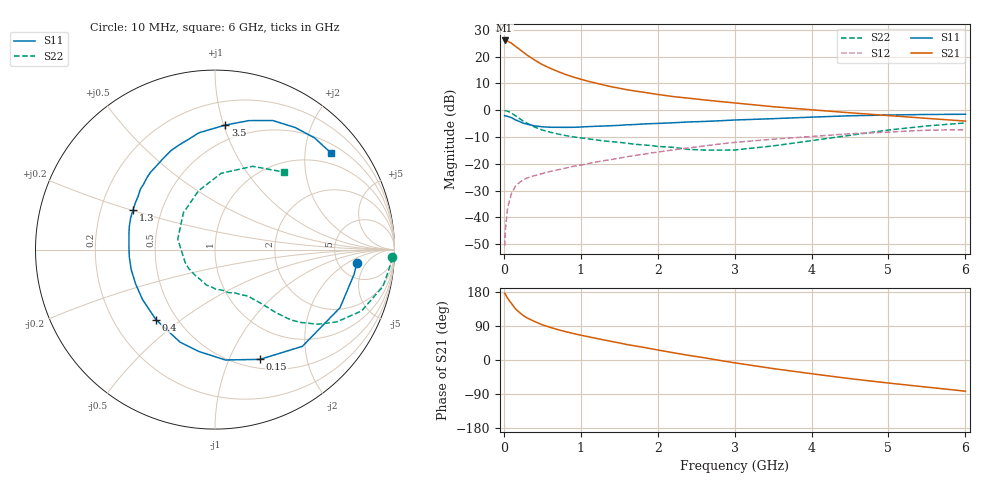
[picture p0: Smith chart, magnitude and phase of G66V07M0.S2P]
! SIEMENS Small Signal Semiconductors
! BFG193
! Si NPN RF Bipolar Junction Transistor in SOT223
! VCE = 6 V  IC = 7 mA
! Common Emitter S-Parameters:  August  1996
# GHz  S  MA  R  50
!  f  S11  S21  S12  S22
! GHz  MAG  ANG  MAG  ANG  MAG  ANG  MAG  ANG
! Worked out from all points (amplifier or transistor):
!   36 points, 10 MHz to 6 GHz, reference 50 ohm
!   highest |S21| = 26.0 dB at 10 MHz (marker M1)
!   |S21| within 3 dB of that: start of sweep to 189.6 MHz
!   unconditionally stable (mu >= 1): 1.019 GHz to 2.538 GHz
!   at 250 MHz: K = 0.42, MSG = 23.9 dB, |S12| = -26.0 dB
!   at 1.4 GHz: K = 1.08, MAG = 11.9 dB, |S12| = -18.4 dB
!   at 6 GHz: K = 0.86, MSG = 1.6 dB, |S12| = -7.3 dB
!   S11 on the Smith chart (normalised r, x): 10 MHz: 7.51, -2.98; 150 MHz: 0.60, -1.31; 400 MHz: 0.39, -0.41; 1.3 GHz: 0.34, +0.20; 3.5 GHz: 0.38, +1.01; 6 GHz: 0.70, +2.58
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0.01  0.7941 -5.3  20.07 176.1  0.0029 87.8  0.9879 -2.5
0.02  0.7869 -10.1  19.96 173.6  0.0059 84.0  0.9811 -5.0
0.05  0.7682 -24.9  19.45 162.4  0.0153 77.5  0.9584 -12.3
0.1  0.7263 -47.9  17.82 148.8  0.0281 68.0  0.8854 -22.7
0.15  0.661 -67.7  15.62 135.3  0.0379 59.2  0.789 -30.7
0.2  0.6178 -84.6  13.85 126.0  0.0444 54.6  0.7075 -36.0
0.25  0.5746 -99.1  12.17 117.8  0.05 50.2  0.6294 -40.2
0.3  0.5511 -110.7  10.75 111.3  0.0541 48.1  0.575 -42.9
0.4  0.5104 -130.2  8.641 101.5  0.0602 45.4  0.4853 -46.1
0.5  0.4905 -145.3  7.117 92.9  0.0659 44.1  0.427 -48.0
0.6  0.4821 -156.4  6.094 86.3  0.0717 44.3  0.3898 -49.7
0.7  0.48 -166.7  5.305 80.3  0.0771 44.5  0.3613 -51.5
0.9  0.48 177.4  4.18 70.0  0.0895 44.6  0.319 -54.5
1.1  0.4946 164.9  3.464 61.3  0.1011 44.8  0.2918 -59.8
1.3  0.5073 154.4  2.953 53.0  0.1143 44.2  0.2671 -64.8
1.6  0.5351 141.0  2.415 40.8  0.1353 41.7  0.2422 -75.6
2.2  0.5832 119.9  1.8 19.3  0.1817 34.4  0.2032 -103.6
2.8  0.6348 102.7  1.459 -0.8  0.2336 24.1  0.1803 -143.0
3.5  0.6962 85.3  1.164 -22.6  0.2881 9.0  0.2157 164.1
4.5  0.7878 65.9  0.896 -49.2  0.3639 -11.1  0.3406 105.6
5.5  0.8336 48.3  0.705 -71.6  0.4242 -36.3  0.5091 65.7
6  0.8406 40.0  0.627 -82.3  0.4323 -50.8  0.5792 48.2
